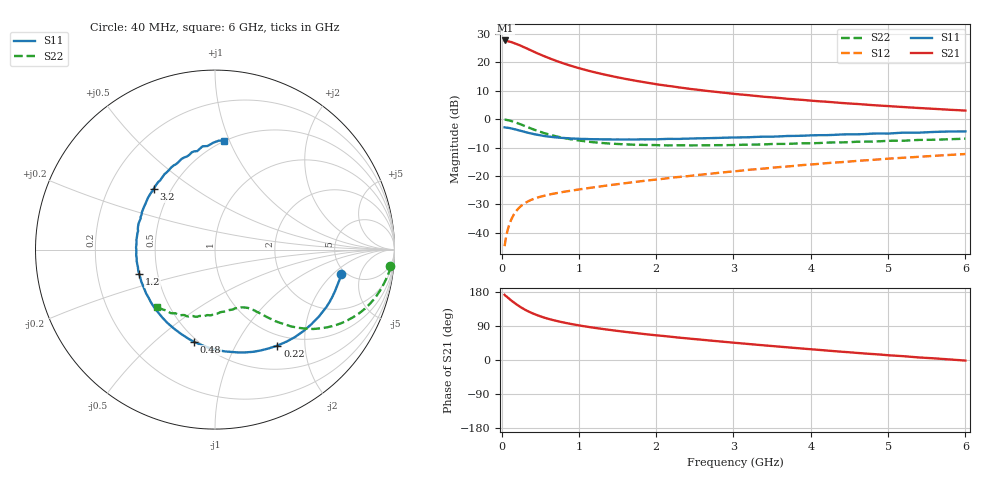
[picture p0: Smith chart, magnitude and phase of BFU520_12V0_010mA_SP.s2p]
! Filename:  P:\Prog\Test\Noise\ATS_data\Testdata_Net\03 Spar\BFU520_APG2013_37_A05_12p0V_010mA_SP_CM01_D.s2p
! Date/Time: Fri 26/Apr/2013 13:00:11
! BFU520_APG2013_37_A05_12p0V_1to20mA_SP_CM01_Bias6_R.s2p
! MDIF S-parameter v. bias file
! BFU520_APG2013_37_A05_12p0V_1to20mA_SP_CM01
! Date/time Tue Apr 23 18:22:57 2013
! VAR V_out= 12.0000
! VAR I_out= 9.9950
! VAR V_in= 0.8100
! VAR I_in= 0.1002
! Device data file deembeded for feedlines and parallel
! Original file: \03 Spar\BFU520_APG2013_37_A05_12p0V_010mA_SP_CM01_R.s2p
! Feed-files: PR047V01_250413_Feed1.s2p, PR047V01_250413_Feed2.s2p
! Parallel-file: PR047V01_250413_Par.s2p
# MHz S MA R 50
!  Freq-MHz  S11-mag  S11-arg  S21-mag  S21-arg  S12-mag  S12-arg  S22-mag  S22-arg
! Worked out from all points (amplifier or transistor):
!   98 points, 40 MHz to 6 GHz, reference 50 ohm
!   highest |S21| = 27.7 dB at 50 MHz (marker M1)
!   |S21| within 3 dB of that: start of sweep to 341.6 MHz
!   unconditionally stable (mu >= 1): 1.877 GHz to 3.885 GHz
!   at 300 MHz: K = 0.30, MSG = 27.4 dB, |S12| = -29.6 dB
!   at 1.6 GHz: K = 0.95, MSG = 18.4 dB, |S12| = -22.5 dB
!   at 6 GHz: K = 0.86, MSG = 7.6 dB, |S12| = -12.3 dB
!   S11 on the Smith chart (normalised r, x): 40 MHz: 4.58, -2.56; 220 MHz: 0.83, -1.50; 480 MHz: 0.48, -0.68; 1.2 GHz: 0.39, -0.13; 3.2 GHz: 0.40, +0.35; 6 GHz: 0.50, +0.96
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40  0.7168 -10.9  24.2 172.0  0.005834 81.9  0.9797 -5.4
50  0.7137 -13.8  24.23 169.5  0.007208 80.8  0.9792 -7.0
120  0.6889 -32.7  22.83 158.1  0.0164 73.8  0.9322 -16.7
140  0.6792 -37.8  22.34 154.8  0.01879 71.6  0.9147 -19.2
180  0.6602 -47.6  21.31 148.8  0.02319 67.6  0.878 -23.9
220  0.6378 -56.9  20.35 143.1  0.02698 64.2  0.8377 -28.0
260  0.6171 -65.6  19.25 137.9  0.03028 61.2  0.7978 -31.7
320  0.5869 -77.5  17.72 131.0  0.03443 57.5  0.7403 -36.3
400  0.5533 -91.2  15.77 123.3  0.03879 53.9  0.6705 -41.0
480  0.5269 -102.9  14.09 116.9  0.04239 51.4  0.6129 -44.6
550  0.5058 -112.2  12.85 111.9  0.04478 50.0  0.5687 -47.0
700  0.4789 -127.8  10.69 103.7  0.04965 48.4  0.5019 -50.8
850  0.4626 -140.4  9.105 97.0  0.05391 48.0  0.4543 -53.5
1050  0.4483 -154.1  7.567 89.7  0.05929 48.4  0.4128 -56.5
1200  0.4436 -162.4  6.701 85.0  0.06337 48.9  0.3916 -58.4
1600  0.4385 179.8  5.117 74.2  0.07474 50.3  0.3605 -63.5
2050  0.4448 165.2  4.025 64.2  0.08801 51.4  0.3478 -70.0
3100  0.4778 136.8  2.711 44.0  0.1243 51.1  0.3538 -86.6
3200  0.4809 135.3  2.639 42.1  0.1286 50.9  0.3563 -87.8
4100  0.5226 115.9  2.066 26.8  0.1633 47.2  0.3796 -103.2
5200  0.5796 96.8  1.633 10.1  0.2097 40.5  0.4175 -121.8
6000  0.6088 85.2  1.416 -1.5  0.2436 34.4  0.4534 -135.1
